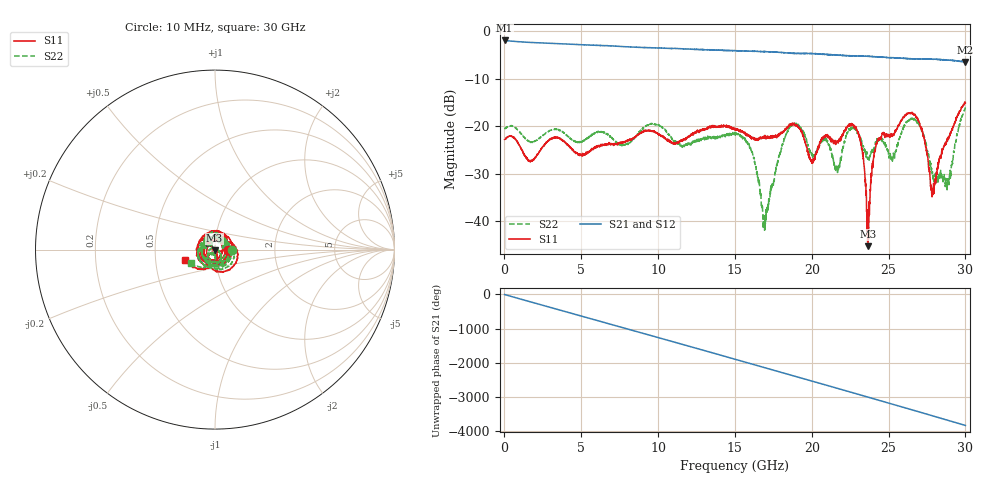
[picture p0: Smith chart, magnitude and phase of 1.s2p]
#  HZ  S  DB  R  50.00
! Rohde & Schwarz Vector Network Analyzer
! Rohde-Schwarz,ZNB40-4Port,1311601084101679,3.45
! Created: UTC 10/20/2022, 5:23:09 PM
! freq[Hz]  db:S11  ang:S11  db:S31  ang:S31  db:S13  ang:S13  db:S33  ang:S33
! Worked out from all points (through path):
!   3000 points, 10 MHz to 30 GHz, reference 50 ohm
!   highest |S21| = -1.96 dB at 10 MHz (marker M1); lowest = -6.5 dB at 29.99 GHz (marker M2)
!   group delay of S21, straight-line fit = 353 ps
!   lowest |S11| = -45.2 dB at 23.67 GHz (marker M3), VSWR 1.01, Z = 49.8 - j0.489 ohm
!   |S11| at or under -10 dB: start of sweep to end of sweep
!   |S22| runs from -41.9 to -16.1 dB; largest |S21 - S12| = 0.01
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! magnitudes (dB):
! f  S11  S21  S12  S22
! 10 MHz  -22.8  -2.0  -2.0  -20.5
! 1.66 GHz  -27.3  -2.4  -2.4  -23.3
! 5.01 GHz  -26.1  -2.9  -2.9  -23.2
! 10.01 GHz  -21.7  -3.5  -3.5  -19.7
! 11.58 GHz  -22.8  -3.7  -3.7  -24.4
! 15.01 GHz  -20.6  -4.1  -4.1  -21.5
! 16.11 GHz  -22.3  -4.2  -4.2  -25.3
! 16.95 GHz  -21.9  -4.3  -4.3  -41.7
! 18.58 GHz  -19.6  -4.6  -4.6  -20.2
! 20.01 GHz  -27.3  -4.7  -4.8  -25.7
! 20.9 GHz  -21.8  -4.9  -4.9  -22.7
! 21.67 GHz  -23.1  -5.0  -5.0  -29.2
! 22.74 GHz  -20.1  -5.2  -5.2  -20.4
! 23.23 GHz  -23.8  -5.3  -5.2  -23.3
! 23.67 GHz  -45.2  -5.3  -5.3  -27.0
! 24.18 GHz  -23.8  -5.4  -5.4  -23.5
! 25.01 GHz  -22.0  -5.6  -5.5  -25.9
! 26.76 GHz  -17.8  -5.8  -5.9  -18.7
! 27.87 GHz  -33.7  -5.9  -5.8  -30.1
! 28.91 GHz  -22.7  -6.1  -6.1  -31.6
! 29.99 GHz  -15.0  -6.5  -6.5  -16.1
! 30 GHz  -15.1  -6.5  -6.4  -16.2
